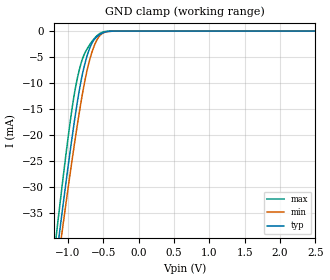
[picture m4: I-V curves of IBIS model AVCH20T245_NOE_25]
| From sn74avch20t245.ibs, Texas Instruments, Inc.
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[Model]   AVCH20T245_NOE_25
Model_type  Input
Vinl=0.7
Vinh=1.6
| variable   typ   min   max
C_comp   2.79pF   2.19pF   3.42pF
[Temperature Range]   40   100   -40
| Ambient temperature   25   85   -40
[Voltage range]   2.5   2.3   2.7
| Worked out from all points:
|   GND clamp passes 1 mA (typ) near -0.58 V on its own axis
[GND Clamp]
| AVCH20T245_NOE_25
|   Voltage   I(typ)   I(min)   I(max)
-4.6V     -459.2mA   -437.9mA   -484.2mA
-1.17V    -44.32mA   -47.52mA   -39.94mA
-1.115V   -38.35mA   -41.89mA   -33.51mA
-1.09V    -35.67mA   -39.36mA   -30.63mA
-1.07V    -33.55mA   -37.35mA   -28.36mA
-945mV    -20.79mA   -25.16mA   -15.18mA
-840mV    -11.44mA   -15.71mA   -7.485mA
-760mV    -6.238mA   -9.522mA   -4.207mA
-685mV    -3.04mA    -5.152mA   -2.477mA
-600mV    -1.199mA   -1.953mA   -1.025mA
-520mV    -424.9uA   -517.7uA   -253uA
2.5V      158.9pA    889.7pA    36.82pA
